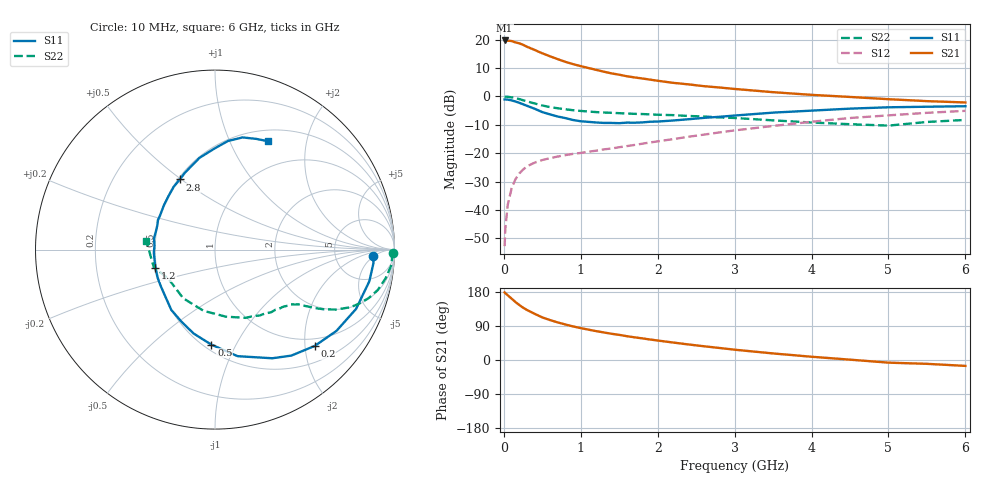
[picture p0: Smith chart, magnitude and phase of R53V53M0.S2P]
! SIEMENS Small Signal Semiconductors
! BFR183
! Si NPN RF Bipolar Junction Transistor in SOT23
! VCE = 3.5 V  IC = 3 mA
! Common Emitter S-Parameters:  May  1996
# GHz  S  MA  R  50
!  f  S11  S21  S12  S22
! GHz  MAG  ANG  MAG  ANG  MAG  ANG  MAG  ANG
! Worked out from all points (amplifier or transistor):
!   36 points, 10 MHz to 6 GHz, reference 50 ohm
!   highest |S21| = 19.7 dB at 10 MHz (marker M1)
!   |S21| within 3 dB of that: start of sweep to 370.3 MHz
!   unconditionally stable (mu >= 1): 1.249 GHz to 2.757 GHz
!   at 250 MHz: K = 0.30, MSG = 22.0 dB, |S12| = -25.8 dB
!   at 1.4 GHz: K = 1.05, MAG = 11.9 dB, |S12| = -18.3 dB
!   at 6 GHz: K = 0.89, MSG = 1.5 dB, |S12| = -5.1 dB
!   lowest NFmin = 1.10 dB at 450 MHz
!   S11 on the Smith chart (normalised r, x): 10 MHz: 14, -5; 200 MHz: 0.83, -2.21; 500 MHz: 0.54, -0.80; 1.2 GHz: 0.49, -0.12; 2.8 GHz: 0.51, +0.49; 6 GHz: 0.64, +1.40
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0.01  0.8827 -2.4  9.685 178.4  0.0023 91.3  0.9934 -1.0
0.02  0.886 -4.9  9.563 176.2  0.0048 85.1  0.9879 -1.9
0.05  0.8778 -11.6  9.596 170.9  0.0122 83.0  0.9872 -4.9
0.1  0.8526 -22.8  9.473 162.2  0.0237 77.3  0.9638 -9.6
0.15  0.8143 -33.8  8.952 153.1  0.0346 72.1  0.9348 -13.9
0.2  0.7726 -44.0  8.63 145.4  0.0438 67.1  0.898 -17.5
0.25  0.7279 -54.2  8.121 138.1  0.0514 62.9  0.857 -20.6
0.3  0.6844 -62.2  7.514 132.1  0.0586 59.7  0.8191 -23.1
0.4  0.6071 -78.0  6.596 121.9  0.0681 54.8  0.7515 -26.4
0.5  0.5298 -92.2  5.753 112.4  0.0757 51.7  0.6931 -28.7
0.6  0.4825 -104.3  5.094 105.4  0.0817 49.8  0.6486 -30.2
0.8  0.4151 -125.9  4.068 93.7  0.0925 48.2  0.5931 -32.0
0.9  0.3841 -135.2  3.707 88.6  0.0972 48.5  0.5719 -32.6
1.1  0.3562 -153.9  3.166 80.1  0.1063 50.1  0.5416 -34.4
1.2  0.3475 -162.8  2.939 76.2  0.1106 50.6  0.5298 -35.2
1.6  0.3455 169.6  2.265 62.8  0.1333 53.1  0.4993 -39.4
2.2  0.3765 139.2  1.736 46.1  0.1768 55.3  0.4683 -48.3
2.8  0.4374 116.6  1.438 31.8  0.2321 53.7  0.4266 -60.4
3.5  0.5184 99.6  1.188 17.3  0.3017 48.1  0.3786 -80.8
4.5  0.6094 83.2  0.979 0.9  0.4167 36.4  0.324 -123.2
5.5  0.6582 69.6  0.826 -10.1  0.5142 22.9  0.3549 -164.2
6  0.672 64.0  0.783 -15.6  0.557 14.2  0.3854 172.9
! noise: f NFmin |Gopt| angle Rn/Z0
0.45  1.1  0.37  35  0.3
0.9  1.15  0.34  85  0.23
1.8  1.9  0.35  160  0.13
